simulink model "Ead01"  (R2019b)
settings: Solver=FixedStepDiscrete  StartTime=0.0  StopTime=10  FixedStep=1  RelTol=1e-3

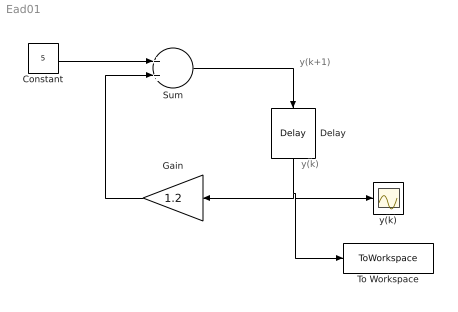
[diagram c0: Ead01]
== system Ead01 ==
  note: y(k+1)
  note: y(k)
  Constant : Constant  Value=5  SampleTime=-1
  Delay : Delay  DelayLength=1  InitialCondition=10
  Gain : Gain  Gain=1.2
  Sum : Sum
  To Workspace : ToWorkspace  VariableName=y  SaveFormat=Timeseries  SampleTime=-1
  y(k) : Scope
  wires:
  Constant/1 -> Sum/1
  Sum/1 -> Delay/1
  Gain/1 -> Sum/2
  Delay/1 -> To Workspace/1, y(k)/1, Gain/1
